| Texas Instruments Incorporated
| TX7332 Three-Level, 32-Channel Transmitter With 1.2-A Pulser, T/R Switch,
| and Integrated Transmit Beamformer
[IBIS Ver]   4.1
[File name]   tx7332.ibs
[File Rev]   1.0
[Date]   03/08/2019
[Source]
| Texas Instruments Incorporated.
| Analog-eLab Design Center, HPA
| 12500 TI Blvd
| Dallas, TX -75243
[Notes]   Revision History:
| Rev 1.0: 03/08/2019
| - Initial version of the model
| - Model generated from simulations in SPECTRE
| - C_comp although listed in numerical order of value are
|   obtained from varying PVT conditions. For PVT conditions for
|   each specific value refer the buffer description under
|   respective [Model]. IBIS model user is responsible for using
|   appropriate C_comp to simulate for Signal Integrity.
| - Warnings regarding combined Non-monotonicity of various models have been
|   reviewd and considered minor and can be ignored.
| - Model names with a trailing _1p8 contain the model for 1.8V operation.
|   Model names with a trailing _2p5 contain the model for 2.5V operation.
| - For lvdsin and lvdsin1 models, use suitable (100Ohms, 200Ohms) termination
|   externally, as internal termination is disabled.
| - TX7332ZBX component is for Differential input configuration of BF_CLKP/M and TR_BF_SYNCP/M pins.
| - TX7332ZBX_B component is for Single ended input configuration of BF_CLKP/M and TR_BF_SYNCP/M pins.
[Disclaimer]
| This model is designed as an aid for customers of Texas Instruments.
| TI and its licensors and suppliers make no warranties, either expressed
| or implied, with respect to this  model, including the warranties of
| merchantability or fitness for a particular purpose. The model is
| provided solely on an "as is" basis. The entire risk as to its quality
| and performance is with the customer.
| This model is subject to change without notice. Texas Instruments
| Incorporated is not responsible for updating this model.
[Copyright]
 (C) Copyright 2019 Texas Instruments Incorporated.All rights reserved.
|  Component TX7332ZBX 260-Pin NFBGA -ZBX package
|  Part # TX7332ZBX
[Component]   TX7332ZBX
[Manufacturer]   TI
[Package]   |260 NFBGA - ZBX package
|   typ   min   max
R_pkg   0.05   0.04   0.06
L_pkg   1.0nH   0.8nH   1.2nH
C_pkg   0.2pF   0.16pF   0.24pF
[Pin]   signal_name   model_name   R_pin   L_pin   C_pin
A1   RX_31   NC   NA   NA   NA
A2   RX_32   NC   NA   NA   NA
A3   IN_32_0   input1   NA   NA   NA
A4   IN_24_0   input1   NA   NA   NA
A5   IN_31_0   input1   NA   NA   NA
A6   IN_23_0   input1   NA   NA   NA
A7   AVSS   gnd   NA   NA   NA
A8   AVSS   gnd   NA   NA   NA
A9   AVDDP_5   power   NA   NA   NA
A10   AVDDM_5   power   NA   NA   NA
A11   AVSS   gnd   NA   NA   NA
A12   AVDDP_HV   power   NA   NA   NA
A13   FLOATP_HV_4   NC   NA   NA   NA
B1   RX_29   NC   NA   NA   NA
B2   RX_30   NC   NA   NA   NA
B3   IN_32_1   input1   NA   NA   NA
B4   IN_24_1   input1   NA   NA   NA
B5   IN_31_1   input1   NA   NA   NA
B6   IN_23_1   input1   NA   NA   NA
B7   AVDD_IO   power   NA   NA   NA
B8   AVSS   gnd   NA   NA   NA
B9   OUT_32   NC   NA   NA   NA
B10   OUT_31   NC   NA   NA   NA
B11   AVSS   gnd   NA   NA   NA
B12   AVDDP_HV   power   NA   NA   NA
B13   AVDDP_HV   power   NA   NA   NA
C1   RX_27   NC   NA   NA   NA
C2   RX_28   NC   NA   NA   NA
C3   IN_30_0   input1   NA   NA   NA
C4   IN_22_0   input1   NA   NA   NA
C5   IN_29_0   input1   NA   NA   NA
C6   IN_21_0   input1   NA   NA   NA
C7   AVDD_IO   power   NA   NA   NA
C8   AVSS   gnd   NA   NA   NA
C9   OUT_30   NC   NA   NA   NA
C10   OUT_29   NC   NA   NA   NA
C11   AVSS   gnd   NA   NA   NA
C12   AVSS   gnd   NA   NA   NA
C13   AVSS   gnd   NA   NA   NA
D1   RX_25   NC   NA   NA   NA
D2   RX_26   NC   NA   NA   NA
D3   IN_30_1   input1   NA   NA   NA
D4   IN_22_1   input1   NA   NA   NA
D5   IN_29_1   input1   NA   NA   NA
D6   IN_21_1   input1   NA   NA   NA
D7   TR_EN4   input1   NA   NA   NA
D8   AVSS   gnd   NA   NA   NA
D9   OUT_28   NC   NA   NA   NA
D10   OUT_27   NC   NA   NA   NA
D11   AVSS   gnd   NA   NA   NA
D12   AVDDM_HV   power   NA   NA   NA
D13   FLOATM_HV4   NC   NA   NA   NA
E1   AVDDP_5   power   NA   NA   NA
E2   AVSS   gnd   NA   NA   NA
E3   IN_28_0   input1   NA   NA   NA
E4   IN_20_0   input1   NA   NA   NA
E5   IN_27_0   input1   NA   NA   NA
E6   IN_19_0   input1   NA   NA   NA
E7   TR_EN3   input1   NA   NA   NA
E8   AVSS   gnd   NA   NA   NA
E9   OUT_26   NC   NA   NA   NA
E10   OUT_25   NC   NA   NA   NA
E11   AVSS   gnd   NA   NA   NA
E12   AVDDM_HV   power   NA   NA   NA
E13   AVDDM_HV   power   NA   NA   NA
F1   RX_23   NC   NA   NA   NA
F2   RX_24   NC   NA   NA   NA
F3   IN_28_1   input1   NA   NA   NA
F4   IN_20_1   input1   NA   NA   NA
F5   IN_27_1   input1   NA   NA   NA
F6   IN_19_1   input1   NA   NA   NA
F7   DSEL_1   input   NA   NA   NA
F8   AVSS   gnd   NA   NA   NA
F9   OUT_24   NC   NA   NA   NA
F10   OUT_23   NC   NA   NA   NA
F11   AVSS   gnd   NA   NA   NA
F12   AVDDM_HV   power   NA   NA   NA
F13   AVDDM_HV   power   NA   NA   NA
G1   RX_21   NC   NA   NA   NA
G2   RX_22   NC   NA   NA   NA
G3   IN_26_0   input1   NA   NA   NA
G4   IN_18_0   input1   NA   NA   NA
G5   IN_25_0   input1   NA   NA   NA
G6   IN_17_0   input1   NA   NA   NA
G7   DSEL_0   input   NA   NA   NA
G8   AVSS   gnd   NA   NA   NA
G9   OUT_22   NC   NA   NA   NA
G10   OUT_21   NC   NA   NA   NA
G11   AVSS   gnd   NA   NA   NA
G12   AVDDM_HV   power   NA   NA   NA
G13   FLOATM_HV_2   NC   NA   NA   NA
H1   RX_19   NC   NA   NA   NA
H2   RX_20   NC   NA   NA   NA
H3   IN_26_1   input1   NA   NA   NA
H4   IN_18_1   input1   NA   NA   NA
H5   IN_25_1   input1   NA   NA   NA
H6   IN_17_1   input1   NA   NA   NA
H7   AVSS   gnd   NA   NA   NA
H8   AVSS   gnd   NA   NA   NA
H9   OUT_20   NC   NA   NA   NA
H10   OUT_19   NC   NA   NA   NA
H11   AVSS   gnd   NA   NA   NA
H12   AVSS   gnd   NA   NA   NA
H13   AVSS   gnd   NA   NA   NA
J1   RX_17   NC   NA   NA   NA
J2   RX_18   NC   NA   NA   NA
J3   AVSS   gnd   NA   NA   NA
J4   AVSS   gnd   NA   NA   NA
J5   RESET   input   NA   NA   NA
J6   SEN_GRP2   input2   NA   NA   NA
J7   AVDDP_5   power   NA   NA   NA
J8   AVDDP_5   power   NA   NA   NA
J9   OUT_18   NC   NA   NA   NA
J10   OUT_17   NC   NA   NA   NA
J11   AVSS   gnd   NA   NA   NA
J12   AVDDP_HV   power   NA   NA   NA
J13   AVDDP_HV   power   NA   NA   NA
K1   BIAS_2P5   NC   NA   NA   NA
K2   AVSS   gnd   NA   NA   NA
K3   BF_CLKP   lvdsin   NA   NA   NA
K4   TR_BF_SYNCP   lvdsin1   NA   NA   NA
K5   SDOUT   output   NA   NA   NA
K6   SDATA_GRP2   input1   NA   NA   NA
K7   AVDDP_5   power   NA   NA   NA
K8   AVSS   gnd   NA   NA   NA
K9   AVSS   gnd   NA   NA   NA
K10   AVDDM_5   power   NA   NA   NA
K11   AVDDM_5   power   NA   NA   NA
K12   AVDDP_HV   power   NA   NA   NA
K13   FLOATP_HV_2   NC   NA   NA   NA
L1   BIAS_2P5   NC   NA   NA   NA
L2   AVSS   gnd   NA   NA   NA
L3   BF_CLKM   lvdsin   NA   NA   NA
L4   TR_BF_SYNCM   lvdsin1   NA   NA   NA
L5   RESYNC   input   NA   NA   NA
L6   SDATA_GRP1   input1   NA   NA   NA
L7   AVDDP_5   power   NA   NA   NA
L8   AVSS   gnd   NA   NA   NA
L9   AVSS   gnd   NA   NA   NA
L10   AVDDM_5   power   NA   NA   NA
L11   AVDDM_5   power   NA   NA   NA
L12   AVDDP_HV   power   NA   NA   NA
L13   FLOATP_HV_3   NC   NA   NA   NA
M1   RX_15   NC   NA   NA   NA
M2   RX_16   NC   NA   NA   NA
M3   AVSS   gnd   NA   NA   NA
M4   AVSS   gnd   NA   NA   NA
M5   SCLK   input   NA   NA   NA
M6   SEN_GRP1   input2   NA   NA   NA
M7   AVDDP_5   power   NA   NA   NA
M8   AVDDP_5   power   NA   NA   NA
M9   OUT_16   NC   NA   NA   NA
M10   OUT_15   NC   NA   NA   NA
M11   AVSS   gnd   NA   NA   NA
M12   AVDDP_HV   power   NA   NA   NA
M13   AVDDP_HV   power   NA   NA   NA
N1   RX_13   NC   NA   NA   NA
N2   RX_14   NC   NA   NA   NA
N3   IN_16_0   input1   NA   NA   NA
N4   IN_8_0   input1   NA   NA   NA
N5   IN_15_0   input1   NA   NA   NA
N6   IN_7_0   input1   NA   NA   NA
N7   AVDD_IO   power   NA   NA   NA
N8   AVSS   gnd   NA   NA   NA
N9   OUT_14   NC   NA   NA   NA
N10   OUT_13   NC   NA   NA   NA
N11   AVSS   gnd   NA   NA   NA
N12   AVSS   gnd   NA   NA   NA
N13   AVSS   gnd   NA   NA   NA
P1   RX_11   NC   NA   NA   NA
P2   RX_12   NC   NA   NA   NA
P3   IN_16_1   input1   NA   NA   NA
P4   IN_8_1   input1   NA   NA   NA
P5   IN_15_1   input1   NA   NA   NA
P6   IN_7_1   input1   NA   NA   NA
P7   SHUTZ   od   NA   NA   NA
P8   AVSS   gnd   NA   NA   NA
P9   OUT_12   NC   NA   NA   NA
P10   OUT_11   NC   NA   NA   NA
P11   AVSS   gnd   NA   NA   NA
P12   AVDDM_HV   power   NA   NA   NA
P13   FLOATM_HV_3   NC   NA   NA   NA
R1   RX_9   NC   NA   NA   NA
R2   RX_10   NC   NA   NA   NA
R3   IN_14_0   input1   NA   NA   NA
R4   IN_6_0   input1   NA   NA   NA
R5   IN_13_0   input1   NA   NA   NA
R6   IN_5_0   input1   NA   NA   NA
R7   TR_EN2   input1   NA   NA   NA
R8   AVSS   gnd   NA   NA   NA
R9   OUT_10   NC   NA   NA   NA
R10   OUT_9   NC   NA   NA   NA
R11   AVSS   gnd   NA   NA   NA
R12   AVDDM_HV   power   NA   NA   NA
R13   AVDDM_HV   power   NA   NA   NA
T1   AVDDP_5   power   NA   NA   NA
T2   AVSS   gnd   NA   NA   NA
T3   IN_14_1   input1   NA   NA   NA
T4   IN_6_1   input1   NA   NA   NA
T5   IN_13_1   input1   NA   NA   NA
T6   IN_5_1   input1   NA   NA   NA
T7   TR_EN1   input1   NA   NA   NA
T8   AVSS   gnd   NA   NA   NA
T9   OUT_8   NC   NA   NA   NA
T10   OUT_7   NC   NA   NA   NA
T11   AVSS   gnd   NA   NA   NA
T12   AVDDM_HV   power   NA   NA   NA
T13   AVDDM_HV   power   NA   NA   NA
U1   RX_7   NC   NA   NA   NA
U2   RX_8   NC   NA   NA   NA
U3   IN_12_0   input1   NA   NA   NA
U4   IN_4_0   input1   NA   NA   NA
U5   IN_11_0   input1   NA   NA   NA
U6   IN_3_0   input1   NA   NA   NA
U7   AVSS   gnd   NA   NA   NA
U8   AVSS   gnd   NA   NA   NA
U9   OUT_6   NC   NA   NA   NA
U10   OUT_5   NC   NA   NA   NA
U11   AVSS   gnd   NA   NA   NA
U12   AVDDM_HV   power   NA   NA   NA
U13   FLOATM_HV_1   NC   NA   NA   NA
V1   RX_5   NC   NA   NA   NA
V2   RX_6   NC   NA   NA   NA
V3   IN_12_1   input1   NA   NA   NA
V4   IN_4_1   input1   NA   NA   NA
V5   IN_11_1   input1   NA   NA   NA
V6   IN_3_1   input1   NA   NA   NA
V7   CW_EN   input   NA   NA   NA
V8   AVSS   gnd   NA   NA   NA
V9   OUT_4   NC   NA   NA   NA
V10   OUT_3   NC   NA   NA   NA
V11   AVSS   gnd   NA   NA   NA
V12   AVSS   gnd   NA   NA   NA
V13   AVSS   gnd   NA   NA   NA
W1   RX_3   NC   NA   NA   NA
W2   RX_4   NC   NA   NA   NA
W3   IN_10_0   input1   NA   NA   NA
W4   IN_2_0   input1   NA   NA   NA
W5   IN_9_0   input1   NA   NA   NA
W6   IN_1_0   input1   NA   NA   NA
W7   STDBY   input   NA   NA   NA
W8   AVSS   gnd   NA   NA   NA
W9   OUT_2   NC   NA   NA   NA
W10   OUT_1   NC   NA   NA   NA
W11   AVSS   gnd   NA   NA   NA
W12   AVDDP_HV   power   NA   NA   NA
W13   AVDDP_HV   power   NA   NA   NA
Y1   RX_1   NC   NA   NA   NA
Y2   RX_2   NC   NA   NA   NA
Y3   IN_10_1   input1   NA   NA   NA
Y4   IN_2_1   input1   NA   NA   NA
Y5   IN_9_1   input1   NA   NA   NA
Y6   IN_1_1   input1   NA   NA   NA
Y7   AVSS   gnd   NA   NA   NA
Y8   AVSS   gnd   NA   NA   NA
Y9   AVDDP_5   power   NA   NA   NA
Y10   AVDDM_5   power   NA   NA   NA
Y11   AVSS   gnd   NA   NA   NA
Y12   AVDDP_HV   power   NA   NA   NA
Y13   FLOATP_HV_1   NC   NA   NA   NA
[Diff_pin]   inv_pin   vdiff   tdelay_typ   tdelay_min   tdelay_max
K3   L3   150mV   NA   NA   NA
K4   L4   150mV   NA   NA   NA
|  Component TX7332ZBX_B 260-Pin NFBGA -ZBX package
|  Part # TX7332ZBX
[Component]   TX7332ZBX_B
[Manufacturer]   TI
[Package]   |260 NFBGA - ZBX package
|   typ   min   max
R_pkg   0.05   0.04   0.06
L_pkg   1.0nH   0.8nH   1.2nH
C_pkg   0.2pF   0.16pF   0.24pF
[Pin]   signal_name   model_name   R_pin   L_pin   C_pin
A1   RX_31   NC   NA   NA   NA
A2   RX_32   NC   NA   NA   NA
A3   IN_32_0   input1   NA   NA   NA
A4   IN_24_0   input1   NA   NA   NA
A5   IN_31_0   input1   NA   NA   NA
A6   IN_23_0   input1   NA   NA   NA
A7   AVSS   gnd   NA   NA   NA
A8   AVSS   gnd   NA   NA   NA
A9   AVDDP_5   power   NA   NA   NA
A10   AVDDM_5   power   NA   NA   NA
A11   AVSS   gnd   NA   NA   NA
A12   AVDDP_HV   power   NA   NA   NA
A13   FLOATP_HV_4   NC   NA   NA   NA
B1   RX_29   NC   NA   NA   NA
B2   RX_30   NC   NA   NA   NA
B3   IN_32_1   input1   NA   NA   NA
B4   IN_24_1   input1   NA   NA   NA
B5   IN_31_1   input1   NA   NA   NA
B6   IN_23_1   input1   NA   NA   NA
B7   AVDD_IO   power   NA   NA   NA
B8   AVSS   gnd   NA   NA   NA
B9   OUT_32   NC   NA   NA   NA
B10   OUT_31   NC   NA   NA   NA
B11   AVSS   gnd   NA   NA   NA
B12   AVDDP_HV   power   NA   NA   NA
B13   AVDDP_HV   power   NA   NA   NA
C1   RX_27   NC   NA   NA   NA
C2   RX_28   NC   NA   NA   NA
C3   IN_30_0   input1   NA   NA   NA
C4   IN_22_0   input1   NA   NA   NA
C5   IN_29_0   input1   NA   NA   NA
C6   IN_21_0   input1   NA   NA   NA
C7   AVDD_IO   power   NA   NA   NA
C8   AVSS   gnd   NA   NA   NA
C9   OUT_30   NC   NA   NA   NA
C10   OUT_29   NC   NA   NA   NA
C11   AVSS   gnd   NA   NA   NA
C12   AVSS   gnd   NA   NA   NA
C13   AVSS   gnd   NA   NA   NA
D1   RX_25   NC   NA   NA   NA
D2   RX_26   NC   NA   NA   NA
D3   IN_30_1   input1   NA   NA   NA
D4   IN_22_1   input1   NA   NA   NA
D5   IN_29_1   input1   NA   NA   NA
D6   IN_21_1   input1   NA   NA   NA
D7   TR_EN4   input1   NA   NA   NA
D8   AVSS   gnd   NA   NA   NA
D9   OUT_28   NC   NA   NA   NA
D10   OUT_27   NC   NA   NA   NA
D11   AVSS   gnd   NA   NA   NA
D12   AVDDM_HV   power   NA   NA   NA
D13   FLOATM_HV4   NC   NA   NA   NA
E1   AVDDP_5   power   NA   NA   NA
E2   AVSS   gnd   NA   NA   NA
E3   IN_28_0   input1   NA   NA   NA
E4   IN_20_0   input1   NA   NA   NA
E5   IN_27_0   input1   NA   NA   NA
E6   IN_19_0   input1   NA   NA   NA
E7   TR_EN3   input1   NA   NA   NA
E8   AVSS   gnd   NA   NA   NA
E9   OUT_26   NC   NA   NA   NA
E10   OUT_25   NC   NA   NA   NA
E11   AVSS   gnd   NA   NA   NA
E12   AVDDM_HV   power   NA   NA   NA
E13   AVDDM_HV   power   NA   NA   NA
F1   RX_23   NC   NA   NA   NA
F2   RX_24   NC   NA   NA   NA
F3   IN_28_1   input1   NA   NA   NA
F4   IN_20_1   input1   NA   NA   NA
F5   IN_27_1   input1   NA   NA   NA
F6   IN_19_1   input1   NA   NA   NA
F7   DSEL_1   input   NA   NA   NA
F8   AVSS   gnd   NA   NA   NA
F9   OUT_24   NC   NA   NA   NA
F10   OUT_23   NC   NA   NA   NA
F11   AVSS   gnd   NA   NA   NA
F12   AVDDM_HV   power   NA   NA   NA
F13   AVDDM_HV   power   NA   NA   NA
G1   RX_21   NC   NA   NA   NA
G2   RX_22   NC   NA   NA   NA
G3   IN_26_0   input1   NA   NA   NA
G4   IN_18_0   input1   NA   NA   NA
G5   IN_25_0   input1   NA   NA   NA
G6   IN_17_0   input1   NA   NA   NA
G7   DSEL_0   input   NA   NA   NA
G8   AVSS   gnd   NA   NA   NA
G9   OUT_22   NC   NA   NA   NA
G10   OUT_21   NC   NA   NA   NA
G11   AVSS   gnd   NA   NA   NA
G12   AVDDM_HV   power   NA   NA   NA
G13   FLOATM_HV_2   NC   NA   NA   NA
H1   RX_19   NC   NA   NA   NA
H2   RX_20   NC   NA   NA   NA
H3   IN_26_1   input1   NA   NA   NA
H4   IN_18_1   input1   NA   NA   NA
H5   IN_25_1   input1   NA   NA   NA
H6   IN_17_1   input1   NA   NA   NA
H7   AVSS   gnd   NA   NA   NA
H8   AVSS   gnd   NA   NA   NA
H9   OUT_20   NC   NA   NA   NA
H10   OUT_19   NC   NA   NA   NA
H11   AVSS   gnd   NA   NA   NA
H12   AVSS   gnd   NA   NA   NA
H13   AVSS   gnd   NA   NA   NA
J1   RX_17   NC   NA   NA   NA
J2   RX_18   NC   NA   NA   NA
J3   AVSS   gnd   NA   NA   NA
J4   AVSS   gnd   NA   NA   NA
J5   RESET   input   NA   NA   NA
J6   SEN_GRP2   input2   NA   NA   NA
J7   AVDDP_5   power   NA   NA   NA
J8   AVDDP_5   power   NA   NA   NA
J9   OUT_18   NC   NA   NA   NA
J10   OUT_17   NC   NA   NA   NA
J11   AVSS   gnd   NA   NA   NA
J12   AVDDP_HV   power   NA   NA   NA
J13   AVDDP_HV   power   NA   NA   NA
K1   BIAS_2P5   NC   NA   NA   NA
K2   AVSS   gnd   NA   NA   NA
K3   BF_CLKP   clkp   NA   NA   NA
K4   TR_BF_SYNCP   syncp   NA   NA   NA
K5   SDOUT   output   NA   NA   NA
K6   SDATA_GRP2   input1   NA   NA   NA
K7   AVDDP_5   power   NA   NA   NA
K8   AVSS   gnd   NA   NA   NA
K9   AVSS   gnd   NA   NA   NA
K10   AVDDM_5   power   NA   NA   NA
K11   AVDDM_5   power   NA   NA   NA
K12   AVDDP_HV   power   NA   NA   NA
K13   FLOATP_HV_2   NC   NA   NA   NA
L1   BIAS_2P5   NC   NA   NA   NA
L2   AVSS   gnd   NA   NA   NA
L3   BF_CLKM   NC   NA   NA   NA
L4   TR_BF_SYNCM   NC   NA   NA   NA
L5   RESYNC   input   NA   NA   NA
L6   SDATA_GRP1   input1   NA   NA   NA
L7   AVDDP_5   power   NA   NA   NA
L8   AVSS   gnd   NA   NA   NA
L9   AVSS   gnd   NA   NA   NA
L10   AVDDM_5   power   NA   NA   NA
L11   AVDDM_5   power   NA   NA   NA
L12   AVDDP_HV   power   NA   NA   NA
L13   FLOATP_HV_3   NC   NA   NA   NA
M1   RX_15   NC   NA   NA   NA
M2   RX_16   NC   NA   NA   NA
M3   AVSS   gnd   NA   NA   NA
M4   AVSS   gnd   NA   NA   NA
M5   SCLK   input   NA   NA   NA
M6   SEN_GRP1   input2   NA   NA   NA
M7   AVDDP_5   power   NA   NA   NA
M8   AVDDP_5   power   NA   NA   NA
M9   OUT_16   NC   NA   NA   NA
M10   OUT_15   NC   NA   NA   NA
M11   AVSS   gnd   NA   NA   NA
M12   AVDDP_HV   power   NA   NA   NA
M13   AVDDP_HV   power   NA   NA   NA
N1   RX_13   NC   NA   NA   NA
N2   RX_14   NC   NA   NA   NA
N3   IN_16_0   input1   NA   NA   NA
N4   IN_8_0   input1   NA   NA   NA
N5   IN_15_0   input1   NA   NA   NA
N6   IN_7_0   input1   NA   NA   NA
N7   AVDD_IO   power   NA   NA   NA
N8   AVSS   gnd   NA   NA   NA
N9   OUT_14   NC   NA   NA   NA
N10   OUT_13   NC   NA   NA   NA
N11   AVSS   gnd   NA   NA   NA
N12   AVSS   gnd   NA   NA   NA
N13   AVSS   gnd   NA   NA   NA
P1   RX_11   NC   NA   NA   NA
P2   RX_12   NC   NA   NA   NA
P3   IN_16_1   input1   NA   NA   NA
P4   IN_8_1   input1   NA   NA   NA
P5   IN_15_1   input1   NA   NA   NA
P6   IN_7_1   input1   NA   NA   NA
P7   SHUTZ   od   NA   NA   NA
P8   AVSS   gnd   NA   NA   NA
P9   OUT_12   NC   NA   NA   NA
P10   OUT_11   NC   NA   NA   NA
P11   AVSS   gnd   NA   NA   NA
P12   AVDDM_HV   power   NA   NA   NA
P13   FLOATM_HV_3   NC   NA   NA   NA
R1   RX_9   NC   NA   NA   NA
R2   RX_10   NC   NA   NA   NA
R3   IN_14_0   input1   NA   NA   NA
R4   IN_6_0   input1   NA   NA   NA
R5   IN_13_0   input1   NA   NA   NA
R6   IN_5_0   input1   NA   NA   NA
R7   TR_EN2   input1   NA   NA   NA
R8   AVSS   gnd   NA   NA   NA
R9   OUT_10   NC   NA   NA   NA
R10   OUT_9   NC   NA   NA   NA
R11   AVSS   gnd   NA   NA   NA
R12   AVDDM_HV   power   NA   NA   NA
R13   AVDDM_HV   power   NA   NA   NA
T1   AVDDP_5   power   NA   NA   NA
T2   AVSS   gnd   NA   NA   NA
T3   IN_14_1   input1   NA   NA   NA
T4   IN_6_1   input1   NA   NA   NA
T5   IN_13_1   input1   NA   NA   NA
T6   IN_5_1   input1   NA   NA   NA
T7   TR_EN1   input1   NA   NA   NA
T8   AVSS   gnd   NA   NA   NA
T9   OUT_8   NC   NA   NA   NA
T10   OUT_7   NC   NA   NA   NA
T11   AVSS   gnd   NA   NA   NA
T12   AVDDM_HV   power   NA   NA   NA
T13   AVDDM_HV   power   NA   NA   NA
U1   RX_7   NC   NA   NA   NA
U2   RX_8   NC   NA   NA   NA
U3   IN_12_0   input1   NA   NA   NA
U4   IN_4_0   input1   NA   NA   NA
U5   IN_11_0   input1   NA   NA   NA
U6   IN_3_0   input1   NA   NA   NA
U7   AVSS   gnd   NA   NA   NA
U8   AVSS   gnd   NA   NA   NA
U9   OUT_6   NC   NA   NA   NA
U10   OUT_5   NC   NA   NA   NA
U11   AVSS   gnd   NA   NA   NA
U12   AVDDM_HV   power   NA   NA   NA
U13   FLOATM_HV_1   NC   NA   NA   NA
V1   RX_5   NC   NA   NA   NA
V2   RX_6   NC   NA   NA   NA
V3   IN_12_1   input1   NA   NA   NA
V4   IN_4_1   input1   NA   NA   NA
V5   IN_11_1   input1   NA   NA   NA
V6   IN_3_1   input1   NA   NA   NA
V7   CW_EN   input   NA   NA   NA
V8   AVSS   gnd   NA   NA   NA
V9   OUT_4   NC   NA   NA   NA
V10   OUT_3   NC   NA   NA   NA
V11   AVSS   gnd   NA   NA   NA
V12   AVSS   gnd   NA   NA   NA
V13   AVSS   gnd   NA   NA   NA
W1   RX_3   NC   NA   NA   NA
W2   RX_4   NC   NA   NA   NA
W3   IN_10_0   input1   NA   NA   NA
W4   IN_2_0   input1   NA   NA   NA
W5   IN_9_0   input1   NA   NA   NA
W6   IN_1_0   input1   NA   NA   NA
W7   STDBY   input   NA   NA   NA
W8   AVSS   gnd   NA   NA   NA
W9   OUT_2   NC   NA   NA   NA
W10   OUT_1   NC   NA   NA   NA
W11   AVSS   gnd   NA   NA   NA
W12   AVDDP_HV   power   NA   NA   NA
W13   AVDDP_HV   power   NA   NA   NA
Y1   RX_1   NC   NA   NA   NA
Y2   RX_2   NC   NA   NA   NA
Y3   IN_10_1   input1   NA   NA   NA
Y4   IN_2_1   input1   NA   NA   NA
Y5   IN_9_1   input1   NA   NA   NA
Y6   IN_1_1   input1   NA   NA   NA
Y7   AVSS   gnd   NA   NA   NA
Y8   AVSS   gnd   NA   NA   NA
Y9   AVDDP_5   power   NA   NA   NA
Y10   AVDDM_5   power   NA   NA   NA
Y11   AVSS   gnd   NA   NA   NA
Y12   AVDDP_HV   power   NA   NA   NA
Y13   FLOATP_HV_1   NC   NA   NA   NA
|   Model Selectors
[Model Selector] input
input_1p8   1.8V   digital input
input_2p5   2.5V   digital input
[Model Selector] input1
input1_1p8   1.8V   digital input
input1_2p5   2.5V   digital input
[Model Selector] input2
input2_1p8   1.8V   digital input
input2_2p5   2.5V   digital input
[Model Selector] output
output_1p8   1.8V   digital output
output_2p5   2.5V   digital output
[Model Selector] od
od_1p8   1.8V   digital output_open_drain
od_2p5   2.5V   digital output_open_drain
[Model Selector] clkp
clkp_1p8   1.8V   digital input
clkp_2p5   2.5V   digital input
[Model Selector] syncp
syncp_1p8   1.8V   digital input
syncp_2p5   2.5V   digital input
| Models and submodels in the file (16): input_1p8 (Input), input_2p5 (Input), input1_1p8 (Input), input1_2p5 (Input), input2_1p8 (Input), input2_2p5 (Input), output_1p8 (3-state), output_2p5 (3-state), od_1p8 (Open_drain), od_2p5 (Open_drain), lvdsin (Input), clkp_1p8 (Input), clkp_2p5 (Input), lvdsin1 (Input), syncp_1p8 (Input), syncp_2p5 (Input)
